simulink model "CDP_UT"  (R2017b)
settings: Solver=FixedStepDiscrete  StartTime=0.0  StopTime=10.0  FixedStep=0.01  RelTol=1e-3  EnableMultiTasking=on
undefined symbols (not defined in the file): ASWTYPE_FALSE, ASWTYPE_TRUE, CaCDP_CellTempNTCVoltTable_mV, CaCDP_CellTempTable_C, CaCDP_CMUPCBTempNTCVoltTable_mV, CaCDP_CMUPCBTempTable_C, CbCDP_DiffBusbarTempStateCheck_flg, CbCDP_DiffCellTempStateCheck_flg, CbCDP_DiffCellVoltStateCheck_flg, CbCDP_IgnorUpdateVld_flg, CbCDP_MaxBusbarTempStateCheck_flg, CbCDP_MaxCellTempStateCheck_flg, CbCDP_MaxCellVoltStateCheck_flg, CbCDP_MinBusbarTempStateCheck_flg, CbCDP_MinCellTempStateCheck_flg, CbCDP_MinCellVoltStateCheck_flg, CcCDP_AFETempConfig_numb, CcCDP_AFETempFltThd_C, CcCDP_AFETempFltThdHys_C, CcCDP_BusbarTempRngFltHiThrd_C, CcCDP_BusbarTempRngFltLowThrd_C, CcCDP_CellDiffFltLevel1_mV, CcCDP_CellDiffFltLevel2_mV, CcCDP_CellDiffFltLevel3_mV, CcCDP_CellTempLowerLimit_C, CcCDP_CellTempRngFltHiThrd_C, CcCDP_CellTempRngFltLowThrd_C, CcCDP_CellTempUpperLimit_C, CcCDP_CellVoltConfig_numb, CcCDP_CellVoltLowerLimit_mV, CcCDP_CellVoltRngHiThrd_mV, CcCDP_CellVoltRngLowThrd_mV, CcCDP_CellVoltUpdateThrd_numb, CcCDP_CellVoltUpperLimit_mV, CcCDP_ChrgMaxCellTempFltLv1Thrd_C, CcCDP_ChrgMaxCellTempFltLv2Thrd_C, CcCDP_ChrgMaxCellTempFltLv3Thrd_C, CcCDP_ChrgMaxCellTempReturnDiff_C, CcCDP_ChrgMinCellTempFltLv1Thrd_C, CcCDP_ChrgMinCellTempFltLv2Thrd_C, CcCDP_ChrgMinCellTempFltLv3Thrd_C, CcCDP_ChrgMinCellTempReturnDiff_C, CcCDP_CMUPCBTempConfig_numb, CcCDP_CMUPCBTempFltThd_C, CcCDP_CMUPCBTempFltThdHys_C, CcCDP_DiffBusbarTempFltLevel1Thrd_C, CcCDP_DiffBusbarTempFltLevel2Thrd_C, CcCDP_DiffBusbarTempReturnDifference_C, CcCDP_DiffCellTempFltLevel1Thrd_C, CcCDP_DiffCellTempFltLevel2Thrd_C, CcCDP_DiffCellTempReturnDifference_C, CcCDP_DiffCellVoltReturnDifference_mV, CcCDP_DiffVoltCheckMaxCellTempCondition_C, CcCDP_DiffVoltCheckMaxCellVoltCondition_mV, CcCDP_DiffVoltCheckMinCellTempCondition_C, CcCDP_DiffVoltCheckMinCellVoltCondition_mV, CcCDP_DiffVoltCheckPackCurrCondition_A, CcCDP_MaxAFETempIniVal_C, CcCDP_MaxBusbarTempFltLevel1Thrd_C, CcCDP_MaxBusbarTempFltLevel2Thrd_C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
libraries: AIWAYS_Powertrain_BMS_lib x148, simulink x8
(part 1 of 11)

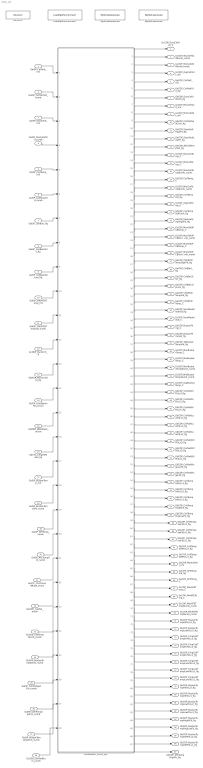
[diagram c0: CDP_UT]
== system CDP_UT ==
  GaISP_CellVolt_mV : Inport
  GaISP_CellVoltVld_numb : Inport  Port=2
  GaISP_StackVolt_mV : Inport  Port=3
  GaISP_StackVoltVld_numb : Inport  Port=4
  GaISP_CellTemp_mV : Inport  Port=5
  GaISP_CellTempVld_numb : Inport  Port=6
  GaISP_CellBalc_flg : Inport  Port=7
  GaISP_CellBalcShrt_flg : Inport  Port=8
  GaISP_CellBalcOpLine_flg : Inport  Port=9
  GaISP_CMUPCBTemp_mV : Inport  Port=10
  GaISP_CMUPCBTempVld_numb : Inport  Port=11
  GcHDP_PackCrnt_A : Inport  Port=12
  GbHDP_PackCrntVld_flg : Inport  Port=13
  GeISP_CmuReIninSts_enum : Inport  Port=14
  GeMSM_BMUState_enum : Inport  Port=15
  GbCTC_ChrgHVMode_flg : Inport  Port=16
  GaISP_BusbarTemp_mV : Inport  Port=17
  GaISP_BusbarTempVld_numb : Inport  Port=18
  GaISP_AFETemp_numb : Inport  Port=19
  GaISP_AFETempVld_numb : Inport  Port=20
  GeCTC_CtrCtlConnMode_enum : Inport  Port=21
  GeUDS_CapSel_enum : Inport  Port=22
  GcUDS_CellTempNumb_numb : Inport  Port=23
  GcUDS_BusbarTempNumb_numb : Inport  Port=24
  GaISP_CellVoltUpdCnt_numb : Inport  Port=25
  GaISP_CellTempUpdCnt_numb : Inport  Port=26
  GaISP_BusbarTempUpdCnt_numb : Inport  Port=27
  GcUDS_CellVoltNum_numb : Inport  Port=28
  CellDataPrc_20ms_sys : Subsystem
  LoadMptEnvironment : AIWAYS_Powertrain_BMS_lib/Config/LoadMptEnvironment  ProjectName=Comm  SuppierID=NewPlatformUAES
  MptA2LGenerate : AIWAYS_Powertrain_BMS_lib/Config/MptA2LGenerate  SystemSampleTime=-1
  MptCodeGenerate : AIWAYS_Powertrain_BMS_lib/Config/MptCodeGenerate  SystemSampleTime=-1
  Revision : AIWAYS_Powertrain_BMS_lib/Config/Revision  curVersion='M110C20'  newVersion='M110C20'
  GcCDP_SumCellVolt_V : Outport
  GcCDP_MaxCellVoltNumb_numb : Outport  Port=2
  GcCDP_MinCellVoltNumb_numb : Outport  Port=3
  GcCDP_AvgCellVolt_mV : Outport  Port=4
  GaCDP_CellVolt_mV : Outport  Port=5
  GaCDP_CellVoltVld_flg : Outport  Port=6
  GbCDP_SumCellVoltVld_flg : Outport  Port=7
  GcCDP_MaxCellVolt_mV : Outport  Port=8
  GcCDP_MinCellVolt_mV : Outport  Port=9
  GbCDP_CellVoltSelfChck_flg : Outport  Port=10
  GaCDP_StackVoltHighFlt_flg : Outport  Port=11
  GaCDP_StackVoltLowFlt_flg : Outport  Port=12
  GbCDP_AllCellTempVld_flg : Outport  Port=13
  GcCDP_MaxCellTemp_C : Outport  Port=14
  GcCDP_MinCellTemp_C : Outport  Port=15
  GcCDP_MaxCellTempNumb_numb : Outport  Port=16
  GaCDP_CellTemp_C : Outport  Port=17
  GcCDP_MinCellTempNumb_numb : Outport  Port=18
  GaCDP_CellTempVld_flg : Outport  Port=19
  GcCDP_AvgCellTemp_C : Outport  Port=20
  GbCDP_CellTempSelfChck_flg : Outport  Port=21
  GaCDP_ModuleTempHighFlt_flg : Outport  Port=22
  GcCDP_MaxCMUPCBTemp_C : Outport  Port=23
  GcCDP_MaxCMUPCBTempNumb_numb : Outport  Port=24
  GcCDP_MinCMUPCBTemp_C : Outport  Port=25
  GcCDP_MinCMUPCBTempNumb_numb : Outport  Port=26
  GbCDP_CMUPCBTempHighFlt_flg : Outport  Port=27
  GaCDP_CellBalc_flg : Outport  Port=28
  GaCDP_CellBalcShrt_flg : Outport  Port=29
  GaCDP_CellBalcOpLine_flg : Outport  Port=30
  GaCDP_CMUPCBTempVld_flg : Outport  Port=31
  GaCDP_CMUPCBTemp_C : Outport  Port=32
  GbCDP_SumModelVoltVld_flg : Outport  Port=33
  GcCDP_SumModelVolt_V : Outport  Port=34
  GaCDP_BusbarTemp_C : Outport  Port=35
  GaCDP_BusbarTempVld_flg : Outport  Port=36
  GbCDP_AllBusbarTempVld_flg : Outport  Port=37
  GcCDP_MaxBusbarTemp_C : Outport  Port=38
  GcCDP_MinBusbarTemp_C : Outport  Port=39
  GcCDP_MaxBusbarTempNumb_numb : Outport  Port=40
  GcCDP_MinBusbarTempNumb_numb : Outport  Port=41
  GcCDP_AvgBusbarTemp_C : Outport  Port=42
  GbCDP_CellVoltHiFltLv3_flg : Outport  Port=43
  GbCDP_CellVoltHiFltLv2_flg : Outport  Port=44
  GbCDP_CellVoltHiFltLv1_flg : Outport  Port=45
  GbCDP_CellVoltLowFltLv3_flg : Outport  Port=46
  GbCDP_CellVoltLowFltLv2_flg : Outport  Port=47
  GbCDP_CellVoltLowFltLv1_flg : Outport  Port=48
  GbCDP_CellVoltDiffFltLv3_flg : Outport  Port=49
  GbCDP_CellVoltDiffFltLv2_flg : Outport  Port=50
  GbCDP_CellVoltDiffFltLv1_flg : Outport  Port=51
  GbCDP_CellVoltRngLowFlt_flg : Outport  Port=52
  GbCDP_CellVoltRngHiFlt_flg : Outport  Port=53
  GbCDP_CellTempHiFltLv3_flg : Outport  Port=54
  GbCDP_CellTempHiFltLv2_flg : Outport  Port=55
  GbCDP_CellTempHiFltLv1_flg : Outport  Port=56
  GbCDP_CellTempRngHiFlt_flg : Outport  Port=57
  GbCDP_CellTempRngLowFlt_flg : Outport  Port=58
  GbCDP_CellTempLowFltLv3_flg : Outport  Port=59
  GbCDP_CellTempLowFltLv2_flg : Outport  Port=60
  GbCDP_CellTempLowFltLv1_flg : Outport  Port=61
  GbCDP_CellTempDiffFltLv2_flg : Outport  Port=62
  GbCDP_CellTempDiffFltLv1_flg : Outport  Port=63
  GaCDP_ModuleVolt_mV : Outport  Port=64
  GaCDP_AFETempVld_flg : Outport  Port=65
  GaCDP_AFETemp_C : Outport  Port=66
  GcCDP_MaxAFETemp_C : Outport  Port=67
  GcCDP_MinAFETemp_C : Outport  Port=68
  GcCDP_MaxAFETempNumb_numb : Outport  Port=69
  GcCDP_MinAFETempNumb_numb : Outport  Port=70
  GbCDP_BusbarTempHiFltLv3_flg : Outport  Port=71
  GbCDP_BusbarTempLowFltLv3_flg : Outport  Port=72
  GbCDP_ChrgCellTempHiFltLv3_flg : Outport  Port=73
  GbCDP_ChrgCellTempHiFltLv2_flg : Outport  Port=74
  GbCDP_ChrgCellTempHiFltLv1_flg : Outport  Port=75
  GbCDP_ChrgCellTempLowFltLv3_flg : Outport  Port=76
  GbCDP_ChrgCellTempLowFltLv2_flg : Outport  Port=77
  GbCDP_ChrgCellTempLowFltLv1_flg : Outport  Port=78
  GbCDP_BusbarTempHiFltLv2_flg : Outport  Port=79
  GbCDP_BusbarTempHiFltLv1_flg : Outport  Port=80
  GbCDP_BusbarTempLowFltLv2_flg : Outport  Port=81
  GbCDP_BusbarTempLowFltLv1_flg : Outport  Port=82
  GbCDP_BusbarTempRngHiFlt_flg : Outport  Port=83
  GbCDP_BusbarTempRngLowFlt_flg : Outport  Port=84
  GbCDP_BusbarTempDiffFltLv2_flg : Outport  Port=85
  GbCDP_BusbarTempDiffFltLv1_flg : Outport  Port=86
  GbCDP_AFETempHighFlt_flg : Outport  Port=87
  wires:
  GaISP_CellVolt_mV/1 -> CellDataPrc_20ms_sys/1(GaISP_CellVolt_mV)
  GaISP_CellVoltVld_numb/1 -> CellDataPrc_20ms_sys/2(GaISP_CellVoltVld_numb)
  GaISP_StackVolt_mV/1 -> CellDataPrc_20ms_sys/3(GaISP_StackVolt_mV)
  GaISP_StackVoltVld_numb/1 -> CellDataPrc_20ms_sys/4(GaISP_StackVoltVld_numb)
  GaISP_CellTemp_mV/1 -> CellDataPrc_20ms_sys/5(GaISP_CellTemp_mV)
  GaISP_CellTempVld_numb/1 -> CellDataPrc_20ms_sys/6(GaISP_CellTempVld_numb)
  GaISP_CellBalc_flg/1 -> CellDataPrc_20ms_sys/7(GaISP_CellBalc_flg)
  GaISP_CellBalcShrt_flg/1 -> CellDataPrc_20ms_sys/8(GaISP_CellBalcShrt_flg)
  GaISP_CellBalcOpLine_flg/1 -> CellDataPrc_20ms_sys/9(GaISP_CellBalcOpLine_flg)
  GaISP_CMUPCBTemp_mV/1 -> CellDataPrc_20ms_sys/10(GaISP_CMUPCBTemp_mV)
  GaISP_CMUPCBTempVld_numb/1 -> CellDataPrc_20ms_sys/11(GaISP_CMUPCBTempVld_numb)
  GcHDP_PackCrnt_A/1 -> CellDataPrc_20ms_sys/12(GcHDP_PackCrnt_A)
  GbHDP_PackCrntVld_flg/1 -> CellDataPrc_20ms_sys/13(GbHDP_PackCrntVld_flg)
  GeISP_CmuReIninSts_enum/1 -> CellDataPrc_20ms_sys/14(GeISP_CmuReIninSts_enum)
  GeMSM_BMUState_enum/1 -> CellDataPrc_20ms_sys/15(GeMSM_BMUState_enum)
  GbCTC_ChrgHVMode_flg/1 -> CellDataPrc_20ms_sys/16(GbCTC_ChrgHVMode_flg)
  GaISP_BusbarTemp_mV/1 -> CellDataPrc_20ms_sys/17(GaISP_BusbarTemp_mV)
  GaISP_BusbarTempVld_numb/1 -> CellDataPrc_20ms_sys/18(GaISP_BusbarTempVld_numb)
  CellDataPrc_20ms_sys/1(GcCDP_SumCellVolt_V) -> GcCDP_SumCellVolt_V/1
  CellDataPrc_20ms_sys/2(GcCDP_MaxCellVoltNumb_numb) -> GcCDP_MaxCellVoltNumb_numb/1
  CellDataPrc_20ms_sys/3(GcCDP_MinCellVoltNumb_numb) -> GcCDP_MinCellVoltNumb_numb/1
  CellDataPrc_20ms_sys/4(GcCDP_AvgCellVolt_mV) -> GcCDP_AvgCellVolt_mV/1
  CellDataPrc_20ms_sys/5(GaCDP_CellVolt_mV) -> GaCDP_CellVolt_mV/1
  CellDataPrc_20ms_sys/6(GaCDP_CellVoltVld_flg) -> GaCDP_CellVoltVld_flg/1
  CellDataPrc_20ms_sys/7(GbCDP_SumCellVoltVld_flg) -> GbCDP_SumCellVoltVld_flg/1
  CellDataPrc_20ms_sys/8(GcCDP_MaxCellVolt_mV) -> GcCDP_MaxCellVolt_mV/1
  CellDataPrc_20ms_sys/9(GcCDP_MinCellVolt_mV) -> GcCDP_MinCellVolt_mV/1
  CellDataPrc_20ms_sys/10(GbCDP_CellVoltSelfChck_flg) -> GbCDP_CellVoltSelfChck_flg/1
  CellDataPrc_20ms_sys/11(GaCDP_StackVoltHighFlt_flg) -> GaCDP_StackVoltHighFlt_flg/1
  CellDataPrc_20ms_sys/12(GaCDP_StackVoltLowFlt_flg) -> GaCDP_StackVoltLowFlt_flg/1
  CellDataPrc_20ms_sys/13(GbCDP_AllCellTempVld_flg) -> GbCDP_AllCellTempVld_flg/1
  CellDataPrc_20ms_sys/14(GcCDP_MaxCellTemp_C) -> GcCDP_MaxCellTemp_C/1
  CellDataPrc_20ms_sys/15(GcCDP_MinCellTemp_C) -> GcCDP_MinCellTemp_C/1
  CellDataPrc_20ms_sys/16(GcCDP_MaxCellTempNumb_numb) -> GcCDP_MaxCellTempNumb_numb/1
  CellDataPrc_20ms_sys/17(GaCDP_CellTemp_C) -> GaCDP_CellTemp_C/1
  CellDataPrc_20ms_sys/18(GcCDP_MinCellTempNumb_numb) -> GcCDP_MinCellTempNumb_numb/1
  CellDataPrc_20ms_sys/19(GaCDP_CellTempVld_flg) -> GaCDP_CellTempVld_flg/1
  CellDataPrc_20ms_sys/20(GcCDP_AvgCellTemp_C) -> GcCDP_AvgCellTemp_C/1
  CellDataPrc_20ms_sys/21(GbCDP_CellTempSelfChck_flg) -> GbCDP_CellTempSelfChck_flg/1
  CellDataPrc_20ms_sys/22(GaCDP_ModuleTempHighFlt_flg) -> GaCDP_ModuleTempHighFlt_flg/1
  CellDataPrc_20ms_sys/23(GcCDP_MaxCMUPCBTemp_C) -> GcCDP_MaxCMUPCBTemp_C/1
  CellDataPrc_20ms_sys/24(GcCDP_MaxCMUPCBTempNumb_numb) -> GcCDP_MaxCMUPCBTempNumb_numb/1
  CellDataPrc_20ms_sys/25(GcCDP_MinCMUPCBTemp_C) -> GcCDP_MinCMUPCBTemp_C/1
  CellDataPrc_20ms_sys/26(GcCDP_MinCMUPCBTempNumb_numb) -> GcCDP_MinCMUPCBTempNumb_numb/1
  CellDataPrc_20ms_sys/27(GbCDP_CMUPCBTempHighFlt_flg) -> GbCDP_CMUPCBTempHighFlt_flg/1
  CellDataPrc_20ms_sys/28(GaCDP_CellBalc_flg) -> GaCDP_CellBalc_flg/1
  CellDataPrc_20ms_sys/29(GaCDP_CellBalcShrt_flg) -> GaCDP_CellBalcShrt_flg/1
  CellDataPrc_20ms_sys/30(GaCDP_CellBalcOpLine_flg) -> GaCDP_CellBalcOpLine_flg/1
  CellDataPrc_20ms_sys/31(GaCDP_CMUPCBTempVld_flg) -> GaCDP_CMUPCBTempVld_flg/1
  CellDataPrc_20ms_sys/32(GaCDP_CMUPCBTemp_C) -> GaCDP_CMUPCBTemp_C/1
  CellDataPrc_20ms_sys/33(GbCDP_SumModelVoltVld_flg) -> GbCDP_SumModelVoltVld_flg/1
  CellDataPrc_20ms_sys/34(GcCDP_SumModelVolt_V) -> GcCDP_SumModelVolt_V/1
  CellDataPrc_20ms_sys/35(GaCDP_BusbarTemp_C) -> GaCDP_BusbarTemp_C/1
  CellDataPrc_20ms_sys/36(GaCDP_BusbarTempVld_flg) -> GaCDP_BusbarTempVld_flg/1
  CellDataPrc_20ms_sys/37(GbCDP_AllBusbarTempVld_flg) -> GbCDP_AllBusbarTempVld_flg/1
  CellDataPrc_20ms_sys/38(GcCDP_MaxBusbarTemp_C) -> GcCDP_MaxBusbarTemp_C/1
  CellDataPrc_20ms_sys/39(GcCDP_MinBusbarTemp_C) -> GcCDP_MinBusbarTemp_C/1
  CellDataPrc_20ms_sys/40(GcCDP_MaxBusbarTempNumb_numb) -> GcCDP_MaxBusbarTempNumb_numb/1
  CellDataPrc_20ms_sys/41(GcCDP_MinBusbarTempNumb_numb) -> GcCDP_MinBusbarTempNumb_numb/1
  CellDataPrc_20ms_sys/42(GcCDP_AvgBusbarTemp_C) -> GcCDP_AvgBusbarTemp_C/1
  CellDataPrc_20ms_sys/43(GbCDP_CellVoltHiFltLv3_flg) -> GbCDP_CellVoltHiFltLv3_flg/1
  CellDataPrc_20ms_sys/44(GbCDP_CellVoltHiFltLv2_flg) -> GbCDP_CellVoltHiFltLv2_flg/1
  CellDataPrc_20ms_sys/45(GbCDP_CellVoltHiFltLv1_flg) -> GbCDP_CellVoltHiFltLv1_flg/1
  CellDataPrc_20ms_sys/46(GbCDP_CellVoltLowFltLv3_flg) -> GbCDP_CellVoltLowFltLv3_flg/1
  CellDataPrc_20ms_sys/47(GbCDP_CellVoltLowFltLv2_flg) -> GbCDP_CellVoltLowFltLv2_flg/1
  CellDataPrc_20ms_sys/48(GbCDP_CellVoltLowFltLv1_flg) -> GbCDP_CellVoltLowFltLv1_flg/1
  CellDataPrc_20ms_sys/49(GbCDP_CellVoltDiffFltLv3_flg) -> GbCDP_CellVoltDiffFltLv3_flg/1
  CellDataPrc_20ms_sys/50(GbCDP_CellVoltDiffFltLv2_flg) -> GbCDP_CellVoltDiffFltLv2_flg/1
  CellDataPrc_20ms_sys/51(GbCDP_CellVoltDiffFltLv1_flg) -> GbCDP_CellVoltDiffFltLv1_flg/1
  CellDataPrc_20ms_sys/52(GbCDP_CellVoltRngLowFlt_flg) -> GbCDP_CellVoltRngLowFlt_flg/1
  CellDataPrc_20ms_sys/53(GbCDP_CellVoltRngHiFlt_flg) -> GbCDP_CellVoltRngHiFlt_flg/1
  CellDataPrc_20ms_sys/54(GbCDP_CellTempHiFltLv3_flg) -> GbCDP_CellTempHiFltLv3_flg/1
  CellDataPrc_20ms_sys/55(GbCDP_CellTempHiFltLv2_flg) -> GbCDP_CellTempHiFltLv2_flg/1
  CellDataPrc_20ms_sys/56(GbCDP_CellTempHiFltLv1_flg) -> GbCDP_CellTempHiFltLv1_flg/1
  CellDataPrc_20ms_sys/57(GbCDP_CellTempRngHiFlt_flg) -> GbCDP_CellTempRngHiFlt_flg/1
  CellDataPrc_20ms_sys/58(GbCDP_CellTempRngLowFlt_flg) -> GbCDP_CellTempRngLowFlt_flg/1
  CellDataPrc_20ms_sys/59(GbCDP_CellTempLowFltLv3_flg) -> GbCDP_CellTempLowFltLv3_flg/1
  CellDataPrc_20ms_sys/60(GbCDP_CellTempLowFltLv2_flg) -> GbCDP_CellTempLowFltLv2_flg/1
  CellDataPrc_20ms_sys/61(GbCDP_CellTempLowFltLv1_flg) -> GbCDP_CellTempLowFltLv1_flg/1
  CellDataPrc_20ms_sys/62(GbCDP_CellTempDiffFltLv2_flg) -> GbCDP_CellTempDiffFltLv2_flg/1
  CellDataPrc_20ms_sys/63(GbCDP_CellTempDiffFltLv1_flg) -> GbCDP_CellTempDiffFltLv1_flg/1
  CellDataPrc_20ms_sys/64(GaCDP_ModuleVolt_mV) -> GaCDP_ModuleVolt_mV/1
  CellDataPrc_20ms_sys/65(GaCDP_AFETempVld_flg) -> GaCDP_AFETempVld_flg/1
  CellDataPrc_20ms_sys/66(GaCDP_AFETemp_C) -> GaCDP_AFETemp_C/1
  CellDataPrc_20ms_sys/67(GcCDP_MaxAFETemp_C) -> GcCDP_MaxAFETemp_C/1
  CellDataPrc_20ms_sys/68(GcCDP_MinAFETemp_C) -> GcCDP_MinAFETemp_C/1
  CellDataPrc_20ms_sys/69(GcCDP_MaxAFETempNumb_numb) -> GcCDP_MaxAFETempNumb_numb/1
  CellDataPrc_20ms_sys/70(GcCDP_MinAFETempNumb_numb) -> GcCDP_MinAFETempNumb_numb/1
  GaISP_AFETemp_numb/1 -> CellDataPrc_20ms_sys/19(GaISP_AFETemp_numb)
  GaISP_AFETempVld_numb/1 -> CellDataPrc_20ms_sys/20(GaISP_AFETempVld_numb)
  CellDataPrc_20ms_sys/71(GbCDP_BusbarTempHiFltLv3_flg) -> GbCDP_BusbarTempHiFltLv3_flg/1
  CellDataPrc_20ms_sys/72(GbCDP_BusbarTempLowFltLv3_flg) -> GbCDP_BusbarTempLowFltLv3_flg/1
  CellDataPrc_20ms_sys/73(GbCDP_ChrgCellTempHiFltLv3_flg) -> GbCDP_ChrgCellTempHiFltLv3_flg/1
  CellDataPrc_20ms_sys/78(GbCDP_ChrgCellTempLowFltLv1_flg) -> GbCDP_ChrgCellTempLowFltLv1_flg/1
  CellDataPrc_20ms_sys/77(GbCDP_ChrgCellTempLowFltLv2_flg) -> GbCDP_ChrgCellTempLowFltLv2_flg/1
  CellDataPrc_20ms_sys/76(GbCDP_ChrgCellTempLowFltLv3_flg) -> GbCDP_ChrgCellTempLowFltLv3_flg/1
  CellDataPrc_20ms_sys/75(GbCDP_ChrgCellTempHiFltLv1_flg) -> GbCDP_ChrgCellTempHiFltLv1_flg/1
  CellDataPrc_20ms_sys/74(GbCDP_ChrgCellTempHiFltLv2_flg) -> GbCDP_ChrgCellTempHiFltLv2_flg/1
  GeCTC_CtrCtlConnMode_enum/1 -> CellDataPrc_20ms_sys/21(GeCTC_CtrCtlConnMode_enum)
  GeUDS_CapSel_enum/1 -> CellDataPrc_20ms_sys/22(GeUDS_CapSel_enum)
  GcUDS_CellTempNumb_numb/1 -> CellDataPrc_20ms_sys/23(GcUDS_CellTempNumb_numb)
  GcUDS_BusbarTempNumb_numb/1 -> CellDataPrc_20ms_sys/24(GcUDS_BusbarTempNumb_numb)
  CellDataPrc_20ms_sys/80(GbCDP_BusbarTempHiFltLv1_flg) -> GbCDP_BusbarTempHiFltLv1_flg/1
  CellDataPrc_20ms_sys/79(GbCDP_BusbarTempHiFltLv2_flg) -> GbCDP_BusbarTempHiFltLv2_flg/1
  CellDataPrc_20ms_sys/81(GbCDP_BusbarTempLowFltLv2_flg) -> GbCDP_BusbarTempLowFltLv2_flg/1
  CellDataPrc_20ms_sys/82(GbCDP_BusbarTempLowFltLv1_flg) -> GbCDP_BusbarTempLowFltLv1_flg/1
  CellDataPrc_20ms_sys/83(GbCDP_BusbarTempRngHiFlt_flg) -> GbCDP_BusbarTempRngHiFlt_flg/1
  CellDataPrc_20ms_sys/84(GbCDP_BusbarTempRngLowFlt_flg) -> GbCDP_BusbarTempRngLowFlt_flg/1
  CellDataPrc_20ms_sys/85(GbCDP_BusbarTempDiffFltLv2_flg) -> GbCDP_BusbarTempDiffFltLv2_flg/1
  CellDataPrc_20ms_sys/86(GbCDP_BusbarTempDiffFltLv1_flg) -> GbCDP_BusbarTempDiffFltLv1_flg/1
  CellDataPrc_20ms_sys/87(GbCDP_AFETempHighFlt_flg) -> GbCDP_AFETempHighFlt_flg/1
  GaISP_CellVoltUpdCnt_numb/1 -> CellDataPrc_20ms_sys/25(GaISP_CellVoltUpdCnt_numb)
  GaISP_CellTempUpdCnt_numb/1 -> CellDataPrc_20ms_sys/26(GaISP_CellTempUpdCnt_numb)
  GaISP_BusbarTempUpdCnt_numb/1 -> CellDataPrc_20ms_sys/27(GaISP_BusbarTempUpdCnt_numb)
  GcUDS_CellVoltNum_numb/1 -> CellDataPrc_20ms_sys/28(GcUDS_CellVoltNum_numb)

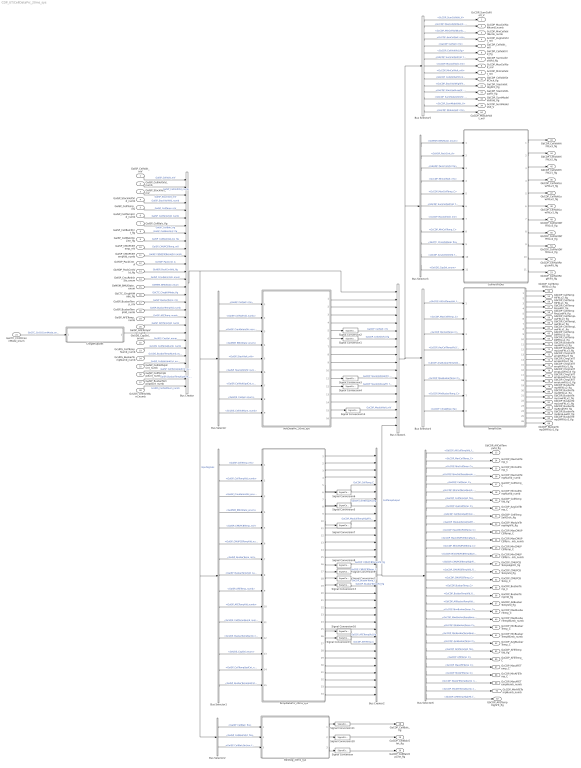
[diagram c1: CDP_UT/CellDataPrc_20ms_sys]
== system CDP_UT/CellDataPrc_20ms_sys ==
  GaISP_CellVolt_mV : Inport
  GaISP_CellVoltVld_numb : Inport  Port=2
  GaISP_StackVolt_mV : Inport  Port=3
  GaISP_StackVoltVld_numb : Inport  Port=4
  GaISP_CellTemp_mV : Inport  Port=5
  GaISP_CellTempVld_numb : Inport  Port=6
  GaISP_CellBalc_flg : Inport  Port=7
  GaISP_CellBalcShrt_flg : Inport  Port=8
  GaISP_CellBalcOpLine_flg : Inport  Port=9
  GaISP_CMUPCBTemp_mV : Inport  Port=10
  GaISP_CMUPCBTempVld_numb : Inport  Port=11
  GcHDP_PackCrnt_A : Inport  Port=12
  GbHDP_PackCrntVld_flg : Inport  Port=13
  GeISP_CmuReIninSts_enum : Inport  Port=14
  GeMSM_BMUState_enum : Inport  Port=15
  GbCTC_ChrgHVMode_flg : Inport  Port=16
  GaISP_BusbarTemp_mV : Inport  Port=17
  GaISP_BusbarTempVld_numb : Inport  Port=18
  GaISP_AFETemp_numb : Inport  Port=19
  GaISP_AFETempVld_numb : Inport  Port=20
  GeCTC_CtrCtlConnMode_enum : Inport  Port=21
  GeUDS_CapSel_enum : Inport  Port=22
  GcUDS_CellTempNumb_numb : Inport  Port=23
  GcUDS_BusbarTempNumb_numb : Inport  Port=24
  GaISP_CellVoltUpdCnt_numb : Inport  Port=25
  GaISP_CellTempUpdCnt_numb : Inport  Port=26
  GaISP_BusbarTempUpdCnt_numb : Inport  Port=27
  GcUDS_CellVoltNum_numb : Inport  Port=28
  BalDiag_20ms_sys : Subsystem
  Bus Creator : BusCreator  Inputs=28
  Bus Creator1 : BusCreator  Inputs=18
  Bus Creator2 : BusCreator  Inputs=34
  Bus Selector : BusSelector  OutputSignals=GaISP_CellVolt_mV,GaISP_CellVoltVld_numb,GeISP_CmuReIninSts_enum,GeMSM_BMUState_enum,GaISP_StackVolt_mV,GaISP_StackVoltVld_numb,GaISP_CellVoltUpdCnt_numb,GeUDS_CapSel_enum,GcUDS_CellVoltNum_numb
  Bus Selector1 : BusSelector  OutputSignals=GaISP_CellTemp_mV,GaISP_CellTempVld_numb,GeISP_CmuReIninSts_enum,GeMSM_BMUState_enum,GaISP_CMUPCBTemp_mV,GaISP_CMUPCBTempVld_numb,GaISP_BusbarTemp_mV,GaISP_BusbarTempVld_numb,GaISP_AFETemp_numb,GaISP_AFETempVld_numb,GcUDS_CellTempNumb_numb,GcUDS_BusbarTempNumb_numb,GeUDS_CapSel_enum,GaISP_CellTempUpdCnt_numb,GaISP_BusbarTempUpdCnt_numb
  Bus Selector2 : BusSelector  OutputSignals=GaISP_CellBalc_flg,GaISP_CellBalcShrt_flg,GaISP_CellBalcOpLine_flg
  Bus Selector3 : BusSelector  OutputSignals=InputSignals.GeMSM_BMUState_enum,InputSignals.GcHDP_PackCrnt_A,InputSignals.GbHDP_PackCrntVld_flg,GcCDP_MinCellVolt_mV,CellTempOutput.GcCDP_MaxCellTemp_C,GbCDP_SumCellVoltVld_flg,GcCDP_MaxCellVolt_mV,CellTempOutput.GcCDP_MinCellTemp_C,InputSignals.GbCTC_ChrgHVMode_flg,LbCDP_AnyCellVoltVld_flg,InputSignals.GeUDS_CapSel_enum
  Bus Selector4 : BusSelector  OutputSignals=CellTempOutput.GbCDP_AllCellTempVld_flg,CellTempOutput.GcCDP_MaxCellTemp_C,CellTempOutput.GcCDP_MinCellTemp_C,CellTempOutput.LbCDP_AnyCellTempVld_flg,CellTempOutput.LbCDP_AnyBusbarTempVld_flg,CellTempOutput.GcCDP_MaxBusbarTemp_C,CellTempOutput.GcCDP_MinBusbarTemp_C,InputSignals.LbCDP_ChrgWkUp_flg
  Bus Selector5 : BusSelector  OutputSignals=GcCDP_SumCellVolt_V,GcCDP_MaxCellVoltNumb_numb,GcCDP_MinCellVoltNumb_numb,GcCDP_AvgCellVolt_mV,GaCDP_CellVolt_mV,GaCDP_CellVoltVld_flg,GbCDP_SumCellVoltVld_flg,GcCDP_MaxCellVolt_mV,GcCDP_MinCellVolt_mV,GbCDP_CellVoltSelfChck_flg,GaCDP_StackVoltHighFlt_flg,GaCDP_StackVoltLowFlt_flg,GbCDP_SumModelVoltVld_flg,GcCDP_SumModelVolt_V,GaCDP_ModuleVolt_mV
  Bus Selector6 : BusSelector  OutputSignals=GbCDP_AllCellTempVld_flg,GcCDP_MaxCellTemp_C,GcCDP_MinCellTemp_C,GcCDP_MaxCellTempNumb_numb,GaCDP_CellTemp_C,GcCDP_MinCellTempNumb_numb,GaCDP_CellTempVld_flg,GcCDP_AvgCellTemp_C,GbCDP_CellTempSelfChck_flg,GaCDP_ModuleTempHighFlt_flg,GcCDP_MaxCMUPCBTemp_C,GcCDP_MaxCMUPCBTempNumb_numb,GcCDP_MinCMUPCBTemp_C,GcCDP_MinCMUPCBTempNumb_numb,GbCDP_CMUPCBTempHighFlt_flg,GaCDP_CMUPCBTempVld_flg,GaCDP_CMUPCBT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
  CellVoltFltDet : Subsystem
  ChrgWkUpDet : Subsystem
  Signal Conversion{,1..16} (17 alike) : SignalConversion  ConversionOutput=Contiguous copy  OverrideOpt=off
  TempDataPrc_20ms_sys : Subsystem
  TempFltDet : Subsystem
  VoltDataPrc_20ms_sys : Subsystem
  GcCDP_SumCellVolt_V : Outport
  GcCDP_MaxCellVoltNumb_numb : Outport  Port=2
  GcCDP_MinCellVoltNumb_numb : Outport  Port=3
  GcCDP_AvgCellVolt_mV : Outport  Port=4
  GaCDP_CellVolt_mV : Outport  Port=5
  GaCDP_CellVoltVld_flg : Outport  Port=6
  GbCDP_SumCellVoltVld_flg : Outport  Port=7
  GcCDP_MaxCellVolt_mV : Outport  Port=8
  GcCDP_MinCellVolt_mV : Outport  Port=9
  GbCDP_CellVoltSelfChck_flg : Outport  Port=10
  GaCDP_StackVoltHighFlt_flg : Outport  Port=11
  GaCDP_StackVoltLowFlt_flg : Outport  Port=12
  GbCDP_AllCellTempVld_flg : Outport  Port=13
  GcCDP_MaxCellTemp_C : Outport  Port=14
  GcCDP_MinCellTemp_C : Outport  Port=15
  GcCDP_MaxCellTempNumb_numb : Outport  Port=16
  GaCDP_CellTemp_C : Outport  Port=17
  GcCDP_MinCellTempNumb_numb : Outport  Port=18
  GaCDP_CellTempVld_flg : Outport  Port=19
  GcCDP_AvgCellTemp_C : Outport  Port=20
  GbCDP_CellTempSelfChck_flg : Outport  Port=21
  GaCDP_ModuleTempHighFlt_flg : Outport  Port=22
  GcCDP_MaxCMUPCBTemp_C : Outport  Port=23
  GcCDP_MaxCMUPCBTempNumb_numb : Outport  Port=24
  GcCDP_MinCMUPCBTemp_C : Outport  Port=25
  GcCDP_MinCMUPCBTempNumb_numb : Outport  Port=26
  GbCDP_CMUPCBTempHighFlt_flg : Outport  Port=27
  GaCDP_CellBalc_flg : Outport  Port=28
  GaCDP_CellBalcShrt_flg : Outport  Port=29
  GaCDP_CellBalcOpLine_flg : Outport  Port=30
  GaCDP_CMUPCBTempVld_flg : Outport  Port=31
  GaCDP_CMUPCBTemp_C : Outport  Port=32
  GbCDP_SumModelVoltVld_flg : Outport  Port=33
  GcCDP_SumModelVolt_V : Outport  Port=34
  GaCDP_BusbarTemp_C : Outport  Port=35
  GaCDP_BusbarTempVld_flg : Outport  Port=36
  GbCDP_AllBusbarTempVld_flg : Outport  Port=37
  GcCDP_MaxBusbarTemp_C : Outport  Port=38
  GcCDP_MinBusbarTemp_C : Outport  Port=39
  GcCDP_MaxBusbarTempNumb_numb : Outport  Port=40
  GcCDP_MinBusbarTempNumb_numb : Outport  Port=41
  GcCDP_AvgBusbarTemp_C : Outport  Port=42
  GbCDP_CellVoltHiFltLv3_flg : Outport  Port=43
  GbCDP_CellVoltHiFltLv2_flg : Outport  Port=44
  GbCDP_CellVoltHiFltLv1_flg : Outport  Port=45
  GbCDP_CellVoltLowFltLv3_flg : Outport  Port=46
  GbCDP_CellVoltLowFltLv2_flg : Outport  Port=47
  GbCDP_CellVoltLowFltLv1_flg : Outport  Port=48
  GbCDP_CellVoltDiffFltLv3_flg : Outport  Port=49
  GbCDP_CellVoltDiffFltLv2_flg : Outport  Port=50
  GbCDP_CellVoltDiffFltLv1_flg : Outport  Port=51
  GbCDP_CellVoltRngLowFlt_flg : Outport  Port=52
  GbCDP_CellVoltRngHiFlt_flg : Outport  Port=53
  GbCDP_CellTempHiFltLv3_flg : Outport  Port=54
  GbCDP_CellTempHiFltLv2_flg : Outport  Port=55
  GbCDP_CellTempHiFltLv1_flg : Outport  Port=56
  GbCDP_CellTempRngHiFlt_flg : Outport  Port=57
  GbCDP_CellTempRngLowFlt_flg : Outport  Port=58
  GbCDP_CellTempLowFltLv3_flg : Outport  Port=59
  GbCDP_CellTempLowFltLv2_flg : Outport  Port=60
  GbCDP_CellTempLowFltLv1_flg : Outport  Port=61
  GbCDP_CellTempDiffFltLv2_flg : Outport  Port=62
  GbCDP_CellTempDiffFltLv1_flg : Outport  Port=63
  GaCDP_ModuleVolt_mV : Outport  Port=64
  GaCDP_AFETempVld_flg : Outport  Port=65
  GaCDP_AFETemp_C : Outport  Port=66
  GcCDP_MaxAFETemp_C : Outport  Port=67
  GcCDP_MinAFETemp_C : Outport  Port=68
  GcCDP_MaxAFETempNumb_numb : Outport  Port=69
  GcCDP_MinAFETempNumb_numb : Outport  Port=70
  GbCDP_BusbarTempHiFltLv3_flg : Outport  Port=71
  GbCDP_BusbarTempLowFltLv3_flg : Outport  Port=72
  GbCDP_ChrgCellTempHiFltLv3_flg : Outport  Port=73
  GbCDP_ChrgCellTempHiFltLv2_flg : Outport  Port=74
  GbCDP_ChrgCellTempHiFltLv1_flg : Outport  Port=75
  GbCDP_ChrgCellTempLowFltLv3_flg : Outport  Port=76
  GbCDP_ChrgCellTempLowFltLv2_flg : Outport  Port=77
  GbCDP_ChrgCellTempLowFltLv1_flg : Outport  Port=78
  GbCDP_BusbarTempHiFltLv2_flg : Outport  Port=79
  GbCDP_BusbarTempHiFltLv1_flg : Outport  Port=80
  GbCDP_BusbarTempLowFltLv2_flg : Outport  Port=81
  GbCDP_BusbarTempLowFltLv1_flg : Outport  Port=82
  GbCDP_BusbarTempRngHiFlt_flg : Outport  Port=83
  GbCDP_BusbarTempRngLowFlt_flg : Outport  Port=84
  GbCDP_BusbarTempDiffFltLv2_flg : Outport  Port=85
  GbCDP_BusbarTempDiffFltLv1_flg : Outport  Port=86
  GbCDP_AFETempHighFlt_flg : Outport  Port=87
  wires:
  Bus Selector/5 -> VoltDataPrc_20ms_sys/5(GaISP_StackVolt_mV)  "<GaISP_StackVolt_mV>"
  Bus Selector/3 -> VoltDataPrc_20ms_sys/3(GeISP_CmuReIninSts_enum)  "<GeISP_CmuReIninSts_enum>"
  Bus Selector6/7 -> GaCDP_CellTempVld_flg/1  "<GaCDP_CellTempVld_flg>"
  Bus Selector6/10 -> GaCDP_ModuleTempHighFlt_flg/1  "<GaCDP_ModuleTempHighFlt_flg>"
  Bus Selector5/3 -> GcCDP_MinCellVoltNumb_numb/1  "<GcCDP_MinCellVoltNumb_numb>"
  GaISP_StackVolt_mV/1 -> Bus Creator/3  "GaISP_StackVolt_mV"
  Bus Selector/1 -> VoltDataPrc_20ms_sys/1(GaISP_CellVolt_mV)  "<GaISP_CellVolt_mV>"
  Bus Selector5/10 -> GbCDP_CellVoltSelfChck_flg/1  "<GbCDP_CellVoltSelfChck_flg>"
  GbCTC_ChrgHVMode_flg/1 -> Bus Creator/16  "GbCTC_ChrgHVMode_flg"
  Bus Selector6/16 -> GaCDP_CMUPCBTempVld_flg/1  "<GaCDP_CMUPCBTempVld_flg>"
  Bus Selector3/3 -> CellVoltFltDet/3(GbHDP_PackCrntVld_flg)  "<GbHDP_PackCrntVld_flg>"
  Bus Selector6/8 -> GcCDP_AvgCellTemp_C/1  "<GcCDP_AvgCellTemp_C>"
  Signal Conversion10/1 -> GaCDP_CellBalcShrt_flg/1
  Bus Selector6/14 -> GcCDP_MinCMUPCBTempNumb_numb/1  "<GcCDP_MinCMUPCBTempNumb_numb>"
  Bus Selector6/12 -> GcCDP_MaxCMUPCBTempNumb_numb/1  "<GcCDP_MaxCMUPCBTempNumb_numb>"
  Bus Selector6/6 -> GcCDP_MinCellTempNumb_numb/1  "<GcCDP_MinCellTempNumb_numb>"
  Bus Selector6/5 -> GaCDP_CellTemp_C/1  "<GaCDP_CellTemp_C>"
  Bus Selector6/4 -> GcCDP_MaxCellTempNumb_numb/1  "<GcCDP_MaxCellTempNumb_numb>"
  Bus Selector6/3 -> GcCDP_MinCellTemp_C/1  "<GcCDP_MinCellTemp_C>"
  Bus Selector5/5 -> GaCDP_CellVolt_mV/1  "<GaCDP_CellVolt_mV>"
  Bus Selector6/2 -> GcCDP_MaxCellTemp_C/1  "<GcCDP_MaxCellTemp_C>"
  Bus Selector5/6 -> GaCDP_CellVoltVld_flg/1  "<GaCDP_CellVoltVld_flg>"
  Signal Conversion/1 -> GaCDP_CellBalcOpLine_flg/1
  Bus Selector3/9 -> CellVoltFltDet/9(GbCTC_ChrgHVMode_flg)  "<GbCTC_ChrgHVMode_flg>"
  Bus Selector3/8 -> CellVoltFltDet/8(GcCDP_MinCellTemp_C)  "<GcCDP_MinCellTemp_C>"
  Bus Selector5/8 -> GcCDP_MaxCellVolt_mV/1  "<GcCDP_MaxCellVolt_mV>"
  Bus Selector6/13 -> GcCDP_MinCMUPCBTemp_C/1  "<GcCDP_MinCMUPCBTemp_C>"
  Bus Selector5/7 -> GbCDP_SumCellVoltVld_flg/1  "<GbCDP_SumCellVoltVld_flg>"
  Bus Selector5/4 -> GcCDP_AvgCellVolt_mV/1  "<GcCDP_AvgCellVolt_mV>"
  Bus Selector5/2 -> GcCDP_MaxCellVoltNumb_numb/1  "<GcCDP_MaxCellVoltNumb_numb>"
  Bus Selector5/1 -> GcCDP_SumCellVolt_V/1  "<GcCDP_SumCellVolt_V>"
  Bus Selector4/3 -> TempFltDet/3(GcCDP_MinCellTemp_C)  "<GcCDP_MinCellTemp_C>"
  Bus Selector3/2 -> CellVoltFltDet/2(GcHDP_PackCrnt_A)  "<GcHDP_PackCrnt_A>"
  Bus Selector3/6 -> CellVoltFltDet/6(GbCDP_SumCellVoltVld_flg)  "<GbCDP_SumCellVoltVld_flg>"
  Bus Selector3/4 -> CellVoltFltDet/4(GcCDP_MinCellVolt_mV)  "<GcCDP_MinCellVolt_mV>"
  Bus Creator2/1 -> Bus Creator1/18, Bus Selector6/1  "CellTempOutput"
  Bus Creator1/1 -> Bus Selector5/1, Bus Selector3/1, Bus Selector4/1
  GaISP_CellBalc_flg/1 -> Bus Creator/7  "GaISP_CellBalc_flg"
  Bus Selector4/2 -> TempFltDet/2(GcCDP_MaxCellTemp_C)  "<GcCDP_MaxCellTemp_C>"
  Bus Selector/4 -> VoltDataPrc_20ms_sys/4(GeMSM_BMUState_enum)  "<GeMSM_BMUState_enum>"
  GeMSM_BMUState_enum/1 -> Bus Creator/15  "GeMSM_BMUState_enum"
  GeISP_CmuReIninSts_enum/1 -> Bus Creator/14  "GeISP_CmuReIninSts_enum"
  GaISP_CMUPCBTempVld_numb/1 -> Bus Creator/11  "GaISP_CMUPCBTempVld_numb"
  Bus Selector5/12 -> GaCDP_StackVoltLowFlt_flg/1  "<GaCDP_StackVoltLowFlt_flg>"
  GbHDP_PackCrntVld_flg/1 -> Bus Creator/13  "GbHDP_PackCrntVld_flg"
  GaISP_CMUPCBTemp_mV/1 -> Bus Creator/10  "GaISP_CMUPCBTemp_mV"
  GaISP_CellBalcOpLine_flg/1 -> Bus Creator/9  "GaISP_CellBalcOpLine_flg"
  GaISP_CellTempVld_numb/1 -> Bus Creator/6  "GaISP_CellTempVld_numb"
  GaISP_CellTemp_mV/1 -> Bus Creator/5  "GaISP_CellTemp_mV"
  Bus Selector5/14 -> GcCDP_SumModelVolt_V/1  "<GcCDP_SumModelVolt_V>"
  Bus Selector6/11 -> GcCDP_MaxCMUPCBTemp_C/1  "<GcCDP_MaxCMUPCBTemp_C>"
  Bus Selector3/1 -> CellVoltFltDet/1(GeMSM_BMUState_enum)  "<GeMSM_BMUState_enum>"
  Bus Selector6/9 -> GbCDP_CellTempSelfChck_flg/1  "<GbCDP_CellTempSelfChck_flg>"
  GcHDP_PackCrnt_A/1 -> Bus Creator/12  "GcHDP_PackCrnt_A"
  Bus Selector4/1 -> TempFltDet/1(GbCDP_AllCellTempVld_flg)  "<GbCDP_AllCellTempVld_flg>"
  Bus Creator/1 -> Bus Selector2/1, Bus Selector1/1, Bus Selector/1, Bus Creator1/1  "InputSignals"
  Bus Selector5/13 -> GbCDP_SumModelVoltVld_flg/1  "<GbCDP_SumModelVoltVld_flg>"
  GaISP_CellVolt_mV/1 -> Bus Creator/1  "GaISP_CellVolt_mV"
  GaISP_CellVoltVld_numb/1 -> Bus Creator/2  "GaISP_CellVoltVld_numb"
  Bus Selector/6 -> VoltDataPrc_20ms_sys/6(GaISP_StackVoltVld_numb)  "<GaISP_StackVoltVld_numb>"
  Bus Selector3/7 -> CellVoltFltDet/7(GcCDP_MaxCellVolt_mV)  "<GcCDP_MaxCellVolt_mV>"
  Bus Selector6/15 -> GbCDP_CMUPCBTempHighFlt_flg/1  "<GbCDP_CMUPCBTempHighFlt_flg>"
  GaISP_CellBalcShrt_flg/1 -> Bus Creator/8  "GaISP_CellBalcShrt_flg"
  Bus Selector/2 -> VoltDataPrc_20ms_sys/2(GaISP_CellVoltVld_numb)  "<GaISP_CellVoltVld_numb>"
  Bus Selector3/5 -> CellVoltFltDet/5(GcCDP_MaxCellTemp_C)  "<GcCDP_MaxCellTemp_C>"
  Bus Selector6/1 -> GbCDP_AllCellTempVld_flg/1  "<GbCDP_AllCellTempVld_flg>"
  Bus Selector5/9 -> GcCDP_MinCellVolt_mV/1  "<GcCDP_MinCellVolt_mV>"
  Bus Selector5/11 -> GaCDP_StackVoltHighFlt_flg/1  "<GaCDP_StackVoltHighFlt_flg>"
  GaISP_StackVoltVld_numb/1 -> Bus Creator/4  "GaISP_StackVoltVld_numb"
  Signal Conversion11/1 -> GaCDP_CellBalc_flg/1
  Bus Selector6/17 -> GaCDP_CMUPCBTemp_C/1  "<GaCDP_CMUPCBTemp_C>"
  VoltDataPrc_20ms_sys/2(GcCDP_MaxCellVoltNumb_numb) -> Bus Creator1/3
  VoltDataPrc_20ms_sys/1(GcCDP_SumCellVolt_V) -> Bus Creator1/2
  VoltDataPrc_20ms_sys/3(GcCDP_MinCellVoltNumb_numb) -> Bus Creator1/4
  VoltDataPrc_20ms_sys/9(GcCDP_MinCellVolt_mV) -> Bus Creator1/10
  VoltDataPrc_20ms_sys/5(GaCDP_CellVolt_mV) -> Signal Conversion2/1
  VoltDataPrc_20ms_sys/4(GcCDP_AvgCellVolt_mV) -> Bus Creator1/5
  VoltDataPrc_20ms_sys/14(GcCDP_SumModelVolt_V) -> Bus Creator1/15
  VoltDataPrc_20ms_sys/8(GcCDP_MaxCellVolt_mV) -> Bus Creator1/9
  VoltDataPrc_20ms_sys/7(GbCDP_SumCellVoltVld_flg) -> Bus Creator1/8
  VoltDataPrc_20ms_sys/13(GbCDP_SumModelVoltVld_flg) -> Bus Creator1/14
  VoltDataPrc_20ms_sys/6(GaCDP_CellVoltVld_flg) -> Signal Conversion1/1
  VoltDataPrc_20ms_sys/11(GaCDP_StackVoltHighFlt_flg) -> Signal Conversion3/1
  VoltDataPrc_20ms_sys/10(GbCDP_CellVoltSelfChck_flg) -> Bus Creator1/11
  VoltDataPrc_20ms_sys/12(GaCDP_StackVoltLowFlt_flg) -> Signal Conversion4/1
  Signal Conversion2/1 -> Bus Creator1/6  "GaCDP_CellVolt_mV"
  Signal Conversion1/1 -> Bus Creator1/7  "GaCDP_CellVoltVld_flg"
  Signal Conversion3/1 -> Bus Creator1/12  "GaCDP_StackVoltHighFlt_flg"
  Signal Conversion4/1 -> Bus Creator1/13  "GaCDP_StackVoltLowFlt_flg"
  TempDataPrc_20ms_sys/3(GcCDP_MinCellTemp_C) -> Bus Creator2/3
  TempDataPrc_20ms_sys/10(GaCDP_ModuleTempHighFlt_flg) -> Signal Conversion7/1
  Signal Conversion6/1 -> Bus Creator2/5  "GaCDP_CellTemp_C"
  TempDataPrc_20ms_sys/12(GcCDP_MaxCMUPCBTempNumb_numb) -> Bus Creator2/12
  Signal Conversion8/1 -> Bus Creator2/16  "GaCDP_CMUPCBTempVld_flg"
  TempDataPrc_20ms_sys/15(GbCDP_CMUPCBTempHighFlt_flg) -> Bus Creator2/15
  Bus Selector1/1 -> TempDataPrc_20ms_sys/1(GaISP_CellTemp_mV)  "<GaISP_CellTemp_mV>"
  Signal Conversion7/1 -> Bus Creator2/10  "GaCDP_ModuleTempHighFlt_flg"
  TempDataPrc_20ms_sys/7(GaCDP_CellTempVld_flg) -> Signal Conversion5/1
  TempDataPrc_20ms_sys/11(GcCDP_MaxCMUPCBTemp_C) -> Bus Creator2/11
  TempDataPrc_20ms_sys/4(GcCDP_MaxCellTempNumb_numb) -> Bus Creator2/4
  TempDataPrc_20ms_sys/1(GbCDP_AllCellTempVld_flg) -> Bus Creator2/1
  TempDataPrc_20ms_sys/13(GcCDP_MinCMUPCBTemp_C) -> Bus Creator2/13
  TempDataPrc_20ms_sys/2(GcCDP_MaxCellTemp_C) -> Bus Creator2/2
  TempDataPrc_20ms_sys/16(GaCDP_CMUPCBTempVld_flg) -> Signal Conversion8/1
  TempDataPrc_20ms_sys/14(GcCDP_MinCMUPCBTempNumb_numb) -> Bus Creator2/14
  Signal Conversion9/1 -> Bus Creator2/17  "GaCDP_CMUPCBTemp_C"
  TempDataPrc_20ms_sys/5(GaCDP_CellTemp_C) -> Signal Conversion6/1
  TempDataPrc_20ms_sys/6(GcCDP_MinCellTempNumb_numb) -> Bus Creator2/6
  Signal Conversion5/1 -> Bus Creator2/7  "GaCDP_CellTempVld_flg"
  TempDataPrc_20ms_sys/8(GcCDP_AvgCellTemp_C) -> Bus Creator2/8
  TempDataPrc_20ms_sys/17(GaCDP_CMUPCBTemp_C) -> Signal Conversion9/1
  Bus Selector1/2 -> TempDataPrc_20ms_sys/2(GaISP_CellTempVld_numb)  "<GaISP_CellTempVld_numb>"
  TempDataPrc_20ms_sys/9(GbCDP_CellTempSelfChck_flg) -> Bus Creator2/9
  Bus Selector1/3 -> TempDataPrc_20ms_sys/3(GeISP_CmuReIninSts_enum)  "<GeISP_CmuReIninSts_enum>"
  Bus Selector1/4 -> TempDataPrc_20ms_sys/4(GeMSM_BMUState_enum)  "<GeMSM_BMUState_enum>"
  Bus Selector1/5 -> TempDataPrc_20ms_sys/5(GaISP_CMUPCBTemp_mV)  "<GaISP_CMUPCBTemp_mV>"
  Bus Selector1/6 -> TempDataPrc_20ms_sys/6(GaISP_CMUPCBTempVld_numb)  "<GaISP_CMUPCBTempVld_numb>"
  Bus Selector2/3 -> BalDiag_20ms_sys/3(GaISP_CellBalcOpLine_flg)  "<GaISP_CellBalcOpLine_flg>"
  BalDiag_20ms_sys/3(GaCDP_CellBalcOpLine_flg) -> Signal Conversion/1
  Bus Selector2/2 -> BalDiag_20ms_sys/2(GaISP_CellBalcShrt_flg)  "<GaISP_CellBalcShrt_flg>"
  Bus Selector2/1 -> BalDiag_20ms_sys/1(GaISP_CellBalc_flg)  "<GaISP_CellBalc_flg>"
  BalDiag_20ms_sys/1(GaCDP_CellBalc_flg) -> Signal Conversion11/1
  BalDiag_20ms_sys/2(GaCDP_CellBalcShrt_flg) -> Signal Conversion10/1
  TempDataPrc_20ms_sys/18(GaCDP_BusbarTemp_C) -> Signal Conversion12/1
  TempDataPrc_20ms_sys/19(GaCDP_BusbarTempVld_flg) -> Signal Conversion13/1
  Signal Conversion12/1 -> Bus Creator2/18  "GaCDP_BusbarTemp_C"
  Signal Conversion13/1 -> Bus Creator2/19  "GaCDP_BusbarTempVld_flg"
  TempDataPrc_20ms_sys/20(GbCDP_AllBusbarTempVld_flg) -> Bus Creator2/20
  TempDataPrc_20ms_sys/21(GcCDP_MaxBusbarTemp_C) -> Bus Creator2/21
  TempDataPrc_20ms_sys/22(GcCDP_MinBusbarTemp_C) -> Bus Creator2/22
  TempDataPrc_20ms_sys/23(GcCDP_MaxBusbarTempNumb_numb) -> Bus Creator2/23
  TempDataPrc_20ms_sys/24(GcCDP_MinBusbarTempNumb_numb) -> Bus Creator2/24
  TempDataPrc_20ms_sys/25(GcCDP_AvgBusbarTemp_C) -> Bus Creator2/25
  Bus Selector6/18 -> GaCDP_BusbarTemp_C/1  "<GaCDP_BusbarTemp_C>"
  Bus Selector6/19 -> GaCDP_BusbarTempVld_flg/1  "<GaCDP_BusbarTempVld_flg>"
  Bus Selector6/20 -> GbCDP_AllBusbarTempVld_flg/1  "<GbCDP_AllBusbarTempVld_flg>"
  Bus Selector6/21 -> GcCDP_MaxBusbarTemp_C/1  "<GcCDP_MaxBusbarTemp_C>"
  Bus Selector6/22 -> GcCDP_MaxBusbarTempNumb_numb/1  "<GcCDP_MaxBusbarTempNumb_numb>"
  Bus Selector6/23 -> GcCDP_MinBusbarTemp_C/1  "<GcCDP_MinBusbarTemp_C>"
  Bus Selector6/24 -> GcCDP_MinBusbarTempNumb_numb/1  "<GcCDP_MinBusbarTempNumb_numb>"
  Bus Selector6/25 -> GcCDP_AvgBusbarTemp_C/1  "<GcCDP_AvgBusbarTemp_C>"
  GaISP_BusbarTemp_mV/1 -> Bus Creator/17  "GaISP_BusbarTemp_mV"
  GaISP_BusbarTempVld_numb/1 -> Bus Creator/18  "GaISP_BusbarTempVld_numb"
  Bus Selector1/7 -> TempDataPrc_20ms_sys/7(GaISP_BusbarTemp_mV)  "<GaISP_BusbarTemp_mV>"
  Bus Selector1/8 -> TempDataPrc_20ms_sys/8(GaISP_BusbarTempVld_numb)  "<GaISP_BusbarTempVld_numb>"
  CellVoltFltDet/1(GbCDP_CellVoltHiFltLv3_flg) -> GbCDP_CellVoltHiFltLv3_flg/1
  CellVoltFltDet/2(GbCDP_CellVoltHiFltLv2_flg) -> GbCDP_CellVoltHiFltLv2_flg/1
  CellVoltFltDet/3(GbCDP_CellVoltHiFltLv1_flg) -> GbCDP_CellVoltHiFltLv1_flg/1
  CellVoltFltDet/4(GbCDP_CellVoltLowFltLv3_flg) -> GbCDP_CellVoltLowFltLv3_flg/1
  CellVoltFltDet/5(GbCDP_CellVoltLowFltLv2_flg) -> GbCDP_CellVoltLowFltLv2_flg/1
  CellVoltFltDet/6(GbCDP_CellVoltLowFltLv1_flg) -> GbCDP_CellVoltLowFltLv1_flg/1
  CellVoltFltDet/7(GbCDP_CellVoltDiffFltLv3_flg) -> GbCDP_CellVoltDiffFltLv3_flg/1
  CellVoltFltDet/8(GbCDP_CellVoltDiffFltLv2_flg) -> GbCDP_CellVoltDiffFltLv2_flg/1
  CellVoltFltDet/9(GbCDP_CellVoltDiffFltLv1_flg) -> GbCDP_CellVoltDiffFltLv1_flg/1
  CellVoltFltDet/10(GbCDP_CellVoltRngLowFlt_flg) -> GbCDP_CellVoltRngLowFlt_flg/1
  CellVoltFltDet/11(GbCDP_CellVoltRngHiFlt_flg) -> GbCDP_CellVoltRngHiFlt_flg/1
  TempFltDet/1(GbCDP_CellTempHiFltLv3_flg) -> GbCDP_CellTempHiFltLv3_flg/1
  TempFltDet/2(GbCDP_CellTempHiFltLv2_flg) -> GbCDP_CellTempHiFltLv2_flg/1
  TempFltDet/3(GbCDP_CellTempHiFltLv1_flg) -> GbCDP_CellTempHiFltLv1_flg/1
  TempFltDet/4(GbCDP_CellTempRngHiFlt_flg) -> GbCDP_CellTempRngHiFlt_flg/1
  TempFltDet/5(GbCDP_CellTempRngLowFlt_flg) -> GbCDP_CellTempRngLowFlt_flg/1
  TempFltDet/6(GbCDP_CellTempLowFltLv3_flg) -> GbCDP_CellTempLowFltLv3_flg/1
  TempFltDet/7(GbCDP_CellTempLowFltLv2_flg) -> GbCDP_CellTempLowFltLv2_flg/1
  TempFltDet/8(GbCDP_CellTempLowFltLv1_flg) -> GbCDP_CellTempLowFltLv1_flg/1
  TempFltDet/9(GbCDP_CellTempDiffFltLv2_flg) -> GbCDP_CellTempDiffFltLv2_flg/1
  TempFltDet/10(GbCDP_CellTempDiffFltLv1_flg) -> GbCDP_CellTempDiffFltLv1_flg/1
  VoltDataPrc_20ms_sys/15(GaCDP_ModuleVolt_mV) -> Signal Conversion14/1
  Bus Selector5/15 -> GaCDP_ModuleVolt_mV/1  "<GaCDP_ModuleVolt_mV>"
  Signal Conversion14/1 -> Bus Creator1/16  "GaCDP_ModuleVolt_mV"
  GaISP_AFETemp_numb/1 -> Bus Creator/19  "GaISP_AFETemp_numb"
  GaISP_AFETempVld_numb/1 -> Bus Creator/20  "GaISP_AFETempVld_numb"
  Bus Selector1/9 -> TempDataPrc_20ms_sys/9(GaISP_AFETemp_numb)  "<GaISP_AFETemp_numb>"
  Bus Selector1/10 -> TempDataPrc_20ms_sys/10(GaISP_AFETempVld_numb)  "<GaISP_AFETempVld_numb>"
  TempDataPrc_20ms_sys/26(GaCDP_AFETempVld_flg) -> Signal Conversion16/1
  TempDataPrc_20ms_sys/27(GaCDP_AFETemp_C) -> Signal Conversion15/1
  Signal Conversion16/1 -> Bus Creator2/26  "GaCDP_AFETempVld_flg"
  Signal Conversion15/1 -> Bus Creator2/27  "GaCDP_AFETemp_C"
  TempDataPrc_20ms_sys/28(GcCDP_MaxAFETemp_C) -> Bus Creator2/28
  TempDataPrc_20ms_sys/29(GcCDP_MinAFETemp_C) -> Bus Creator2/29
  TempDataPrc_20ms_sys/30(GcCDP_MaxAFETempNumb_numb) -> Bus Creator2/30
  TempDataPrc_20ms_sys/31(GcCDP_MinAFETempNumb_numb) -> Bus Creator2/31
  Bus Selector6/26 -> GaCDP_AFETempVld_flg/1  "<GaCDP_AFETempVld_flg>"
  Bus Selector6/27 -> GaCDP_AFETemp_C/1  "<GaCDP_AFETemp_C>"
  Bus Selector6/28 -> GcCDP_MaxAFETemp_C/1  "<GcCDP_MaxAFETemp_C>"
  Bus Selector6/29 -> GcCDP_MinAFETemp_C/1  "<GcCDP_MinAFETemp_C>"
  Bus Selector6/30 -> GcCDP_MaxAFETempNumb_numb/1  "<GcCDP_MaxAFETempNumb_numb>"
  Bus Selector6/31 -> GcCDP_MinAFETempNumb_numb/1  "<GcCDP_MinAFETempNumb_numb>"
  VoltDataPrc_20ms_sys/16(LbCDP_AnyCellVoltVld_flg) -> Bus Creator1/17
  Bus Selector3/10 -> CellVoltFltDet/10(LbCDP_AnyCellVoltVld_flg)  "<LbCDP_AnyCellVoltVld_flg>"
  TempDataPrc_20ms_sys/32(LbCDP_AnyCellTempVld_flg) -> Bus Creator2/32
  Bus Selector4/4 -> TempFltDet/4(LbCDP_AnyCellTempVld_flg)  "<LbCDP_AnyCellTempVld_flg>"
  TempDataPrc_20ms_sys/33(LbCDP_AnyBusbarTempVld_flg) -> Bus Creator2/33
  Bus Selector4/5 -> TempFltDet/5(LbCDP_AnyBusbarTempVld_flg)  "<LbCDP_AnyBusbarTempVld_flg>"
  Bus Selector4/6 -> TempFltDet/6(GcCDP_MaxBusbarTemp_C)  "<GcCDP_MaxBusbarTemp_C>"
  Bus Selector4/7 -> TempFltDet/7(GcCDP_MinBusbarTemp_C)  "<GcCDP_MinBusbarTemp_C>"
  TempFltDet/12(GbCDP_BusbarTempLowFltLv3_flg) -> GbCDP_BusbarTempLowFltLv3_flg/1
  TempFltDet/11(GbCDP_BusbarTempHiFltLv3_flg) -> GbCDP_BusbarTempHiFltLv3_flg/1
  GeCTC_CtrCtlConnMode_enum/1 -> ChrgWkUpDet/1(GeCTC_CtrCtlConnMode_enum)  "GeCTC_CtrCtlConnMode_enum"
  ChrgWkUpDet/1(LbCDP_ChrgWkUp_flg) -> Bus Creator/21
  Bus Selector4/8 -> TempFltDet/8(LbCDP_ChrgWkUp_flg)  "<LbCDP_ChrgWkUp_flg>"
  TempFltDet/13(GbCDP_ChrgCellTempHiFltLv3_flg) -> GbCDP_ChrgCellTempHiFltLv3_flg/1
  TempFltDet/14(GbCDP_ChrgCellTempHiFltLv2_flg) -> GbCDP_ChrgCellTempHiFltLv2_flg/1
  TempFltDet/15(GbCDP_ChrgCellTempHiFltLv1_flg) -> GbCDP_ChrgCellTempHiFltLv1_flg/1
  TempFltDet/16(GbCDP_ChrgCellTempLowFltLv3_flg) -> GbCDP_ChrgCellTempLowFltLv3_flg/1
  TempFltDet/17(GbCDP_ChrgCellTempLowFltLv2_flg) -> GbCDP_ChrgCellTempLowFltLv2_flg/1
  TempFltDet/18(GbCDP_ChrgCellTempLowFltLv1_flg) -> GbCDP_ChrgCellTempLowFltLv1_flg/1
  GeUDS_CapSel_enum/1 -> Bus Creator/22  "GeUDS_CapSel_enum"
  Bus Selector3/11 -> CellVoltFltDet/11(GeUDS_CapSel_enum)  "<GeUDS_CapSel_enum>"
  GcUDS_CellTempNumb_numb/1 -> Bus Creator/23  "GcUDS_CellTempNumb_numb"
  GcUDS_BusbarTempNumb_numb/1 -> Bus Creator/24  "GcUDS_BusbarTempNumb_numb"
  Bus Selector1/11 -> TempDataPrc_20ms_sys/11(GcUDS_CellTempNumb_numb)  "<GcUDS_CellTempNumb_numb>"
  Bus Selector1/12 -> TempDataPrc_20ms_sys/12(GcUDS_BusbarTempNumb_numb)  "<GcUDS_BusbarTempNumb_numb>"
  TempFltDet/19(GbCDP_BusbarTempHiFltLv2_flg) -> GbCDP_BusbarTempHiFltLv2_flg/1
  TempFltDet/20(GbCDP_BusbarTempHiFltLv1_flg) -> GbCDP_BusbarTempHiFltLv1_flg/1
  TempFltDet/21(GbCDP_BusbarTempLowFltLv2_flg) -> GbCDP_BusbarTempLowFltLv2_flg/1
  TempFltDet/22(GbCDP_BusbarTempLowFltLv1_flg) -> GbCDP_BusbarTempLowFltLv1_flg/1
  TempFltDet/23(GbCDP_BusbarTempRngHiFlt_flg) -> GbCDP_BusbarTempRngHiFlt_flg/1
  TempFltDet/24(GbCDP_BusbarTempRngLowFlt_flg) -> GbCDP_BusbarTempRngLowFlt_flg/1
  TempFltDet/25(GbCDP_BusbarTempDiffFltLv2_flg) -> GbCDP_BusbarTempDiffFltLv2_flg/1
  TempFltDet/26(GbCDP_BusbarTempDiffFltLv1_flg) -> GbCDP_BusbarTempDiffFltLv1_flg/1
  TempDataPrc_20ms_sys/34(GbCDP_AFETempHighFlt_flg) -> Bus Creator2/34
  Bus Selector6/32 -> GbCDP_AFETempHighFlt_flg/1  "<GbCDP_AFETempHighFlt_flg>"
  GaISP_CellVoltUpdCnt_numb/1 -> Bus Creator/25  "GaISP_CellVoltUpdCnt_numb"
  Bus Selector/7 -> VoltDataPrc_20ms_sys/7(GaISP_CellVoltUpdCnt_numb)  "<GaISP_CellVoltUpdCnt_numb>"
  Bus Selector/8 -> VoltDataPrc_20ms_sys/8(GeUDS_CapSel_enum)  "<GeUDS_CapSel_enum>"
  Bus Selector1/13 -> TempDataPrc_20ms_sys/13(GeUDS_CapSel_enum)  "<GeUDS_CapSel_enum>"
  Bus Selector1/14 -> TempDataPrc_20ms_sys/14(GaISP_CellTempUpdCnt_numb)  "<GaISP_CellTempUpdCnt_numb>"
  GaISP_CellTempUpdCnt_numb/1 -> Bus Creator/26  "GaISP_CellTempUpdCnt_numb"
  GaISP_BusbarTempUpdCnt_numb/1 -> Bus Creator/27  "GaISP_BusbarTempUpdCnt_numb"
  Bus Selector1/15 -> TempDataPrc_20ms_sys/15(GaISP_BusbarTempUpdCnt_numb)  "<GaISP_BusbarTempUpdCnt_numb>"
  GcUDS_CellVoltNum_numb/1 -> Bus Creator/28  "GcUDS_CellVoltNum_numb"
  Bus Selector/9 -> VoltDataPrc_20ms_sys/9(GcUDS_CellVoltNum_numb)  "<GcUDS_CellVoltNum_numb>"

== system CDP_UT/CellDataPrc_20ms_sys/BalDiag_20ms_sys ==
  GaISP_CellBalc_flg : Inport
  GaISP_CellBalcShrt_flg : Inport  Port=2
  GaISP_CellBalcOpLine_flg : Inport  Port=3
  CDP_GaCDP_CellBalcOpLine_flg : AIWAYS_Powertrain_BMS_lib/Signals/OverWrite  OverWrite_Value=CaCDP_CellBalcOpLineOvr_flg  OverWrite_flag=CbCDP_CellBalcOpLineOvrSwt_flg
  CDP_GaCDP_CellBalcShrt_flg : AIWAYS_Powertrain_BMS_lib/Signals/OverWrite  OverWrite_Value=CaCDP_CellBalcShrtOvr_flg  OverWrite_flag=CbCDP_CellBalcShrtOvrSwt_flg
  CDP_GaCDP_CellBalc_flg : AIWAYS_Powertrain_BMS_lib/Signals/OverWrite  OverWrite_Value=CaCDP_CellBalcOvr_flg  OverWrite_flag=CbCDP_CellBalcOvrSwt_flg
  GaCDP_CellBalc_flg : Outport
  GaCDP_CellBalcShrt_flg : Outport  Port=2
  GaCDP_CellBalcOpLine_flg : Outport  Port=3
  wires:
  GaISP_CellBalc_flg/1 -> CDP_GaCDP_CellBalc_flg/1  "GaISP_CellBalc_flg"
  CDP_GaCDP_CellBalc_flg/1 -> GaCDP_CellBalc_flg/1  "GaCDP_CellBalc_flg"
  GaISP_CellBalcShrt_flg/1 -> CDP_GaCDP_CellBalcShrt_flg/1  "GaISP_CellBalcShrt_flg"
  CDP_GaCDP_CellBalcShrt_flg/1 -> GaCDP_CellBalcShrt_flg/1  "GaCDP_CellBalcShrt_flg"
  GaISP_CellBalcOpLine_flg/1 -> CDP_GaCDP_CellBalcOpLine_flg/1  "GaISP_CellBalcOpLine_flg"
  CDP_GaCDP_CellBalcOpLine_flg/1 -> GaCDP_CellBalcOpLine_flg/1  "GaCDP_CellBalcOpLine_flg"
